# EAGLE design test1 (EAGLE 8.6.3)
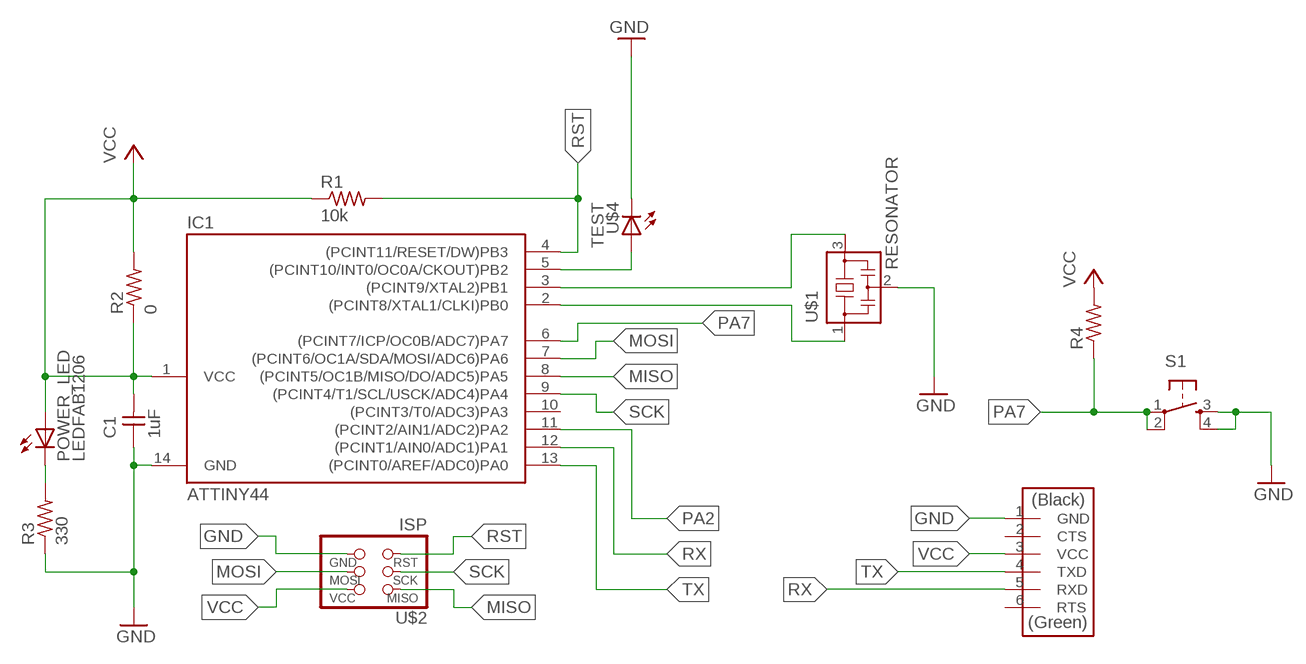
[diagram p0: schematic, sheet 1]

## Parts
C1  1uF  CAP-UNPOLARIZEDFAB  [C1206FAB]
FTDI  FTDI-SMD-HEADER  [1X06SMD]
IC1  ATTINY44  ATTINY44-SSU  [SOIC14]
POWER_LED  LEDFAB1206  [LED1206FAB]
R1  10k  RES-US1206FAB  [R1206FAB]
R2  0  RES-US1206FAB  [R1206FAB]
R3  330  RES-US1206FAB  [R1206FAB]
R4  RES-US1206FAB  [R1206FAB]
S1  6MM_SWITCH6MM_SWITCH  [6MM_SWITCH]
U$1  RESONATOR  [EFOBM]
U$2  ISP  AVRISPSMD  [2X03SMD]
U$4  TEST  LEDFAB1206  [LED1206FAB]

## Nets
GND: C1.1 FTDI.1(GND) IC1.14(GND) R3.1 S1.3(S) S1.4(S1) U$1.2 U$2.6(GND) U$4.2(C)
MISO: IC1.8((PCINT5/OC1B/MISO/DO/ADC5)PA5) U$2.1(MISO)
MOSI: IC1.7((PCINT6/OC1A/SDA/MOSI/ADC6)PA6) U$2.4(MOSI)
N$1: IC1.3((PCINT9/XTAL2)PB1) U$1.3
N$2: IC1.2((PCINT8/XTAL1/CLKI)PB0) U$1.1
N$4: POWER_LED.2(C) R3.2
N$6: IC1.5((PCINT10/INT0/OC0A/CKOUT)PB2) U$4.1(A)
PA2: IC1.11((PCINT2/AIN1/ADC2)PA2)
PA7: IC1.6((PCINT7/ICP/OC0B/ADC7)PA7) R4.1 S1.1(P) S1.2(P1)
RST: IC1.4((PCINT11/RESET/DW)PB3) R1.2 U$2.5(RST)
RX: FTDI.5(RXD) IC1.12((PCINT1/AIN0/ADC1)PA1)
SCK: IC1.9((PCINT4/T1/SCL/USCK/ADC4)PA4) U$2.3(SCK)
TX: FTDI.4(TXD) IC1.13((PCINT0/AREF/ADC0)PA0)
VCC: C1.2 FTDI.3(VCC) IC1.1(VCC) POWER_LED.1(A) R1.1 R2.1 R2.2 R4.2 U$2.2(VCC)
Unconnected: FTDI.2(CTS) FTDI.6(RTS) IC1.10((PCINT3/T0/ADC3)PA3)

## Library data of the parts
C1 = fab:CAP-UNPOLARIZED
FTDI = fab:FTDI-SMD-HEADER
IC1 = fab:ATTINY44
POWER_LED U$4 = fab:LED: LED
R1-R4 = fab:RES-US: Resistor (US Symbol)
S1 = fab:6MM_SWITCH: OMRON SWITCH
U$1 = fab:RESONATOR
U$2 = fab:AVRISP

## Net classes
0 default: width 0.508 mm, clearance 0.152 mm

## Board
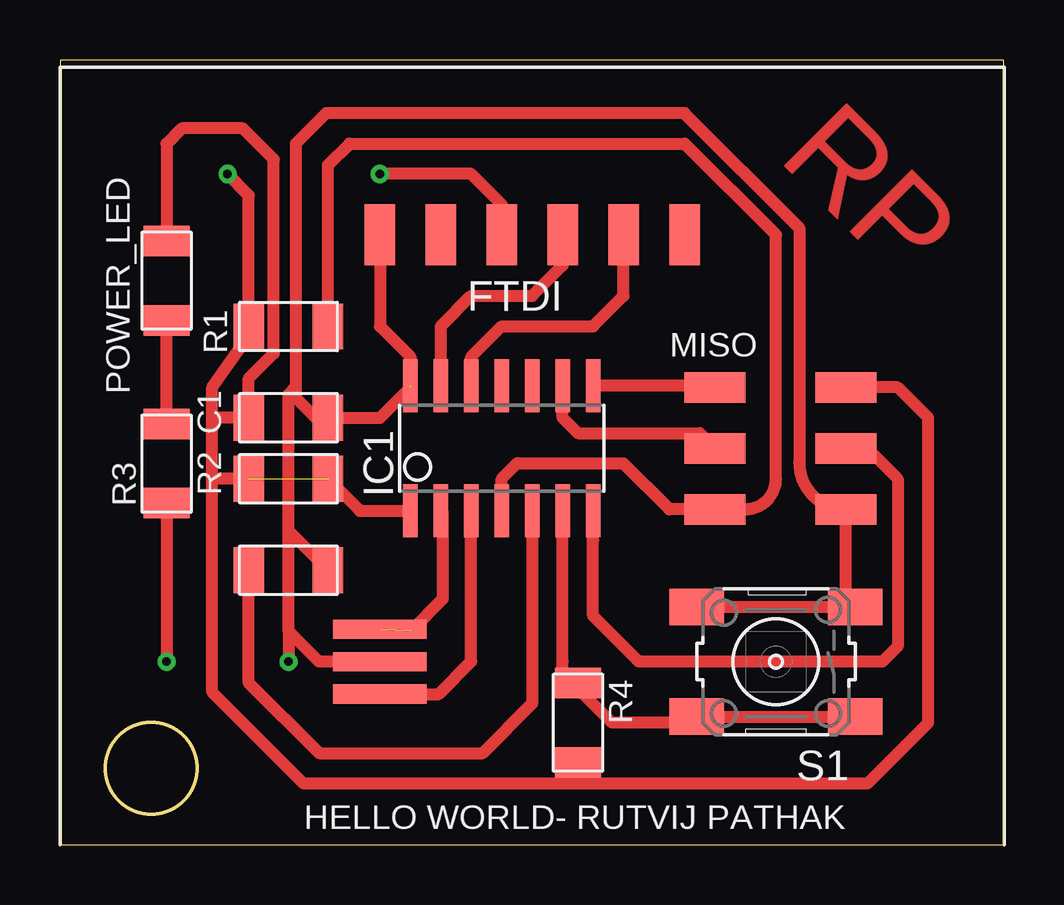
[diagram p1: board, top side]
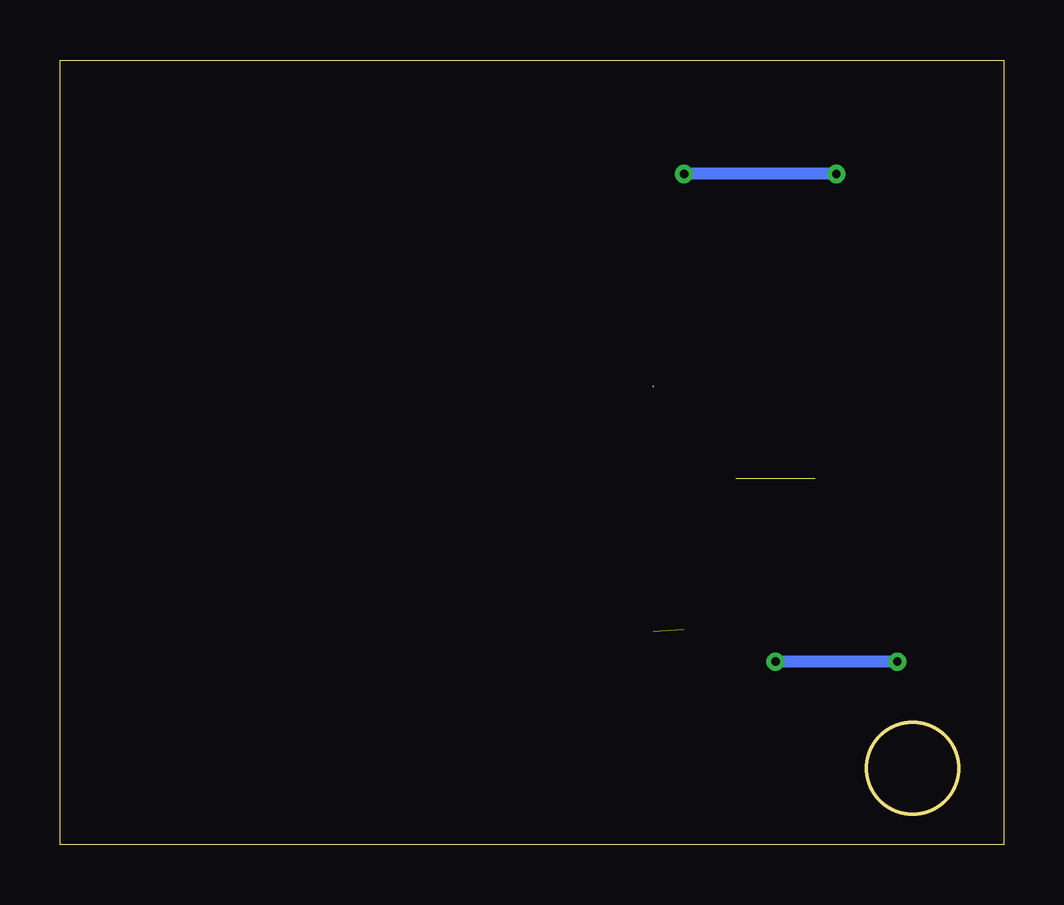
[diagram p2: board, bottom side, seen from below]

Size 39.35 x 32.69 mm. Coordinates in mm from the lower left corner, seen from the top.
Outline: 0,0 39.35,0 39.35,32.69 0,32.69 0,0
Outline: circle at 3.81,3.17 radius 1.91
Copper layers (1*16): Top 0.035mm / dielectric 1.5mm / Bottom 0.035mm
Design rules "default": minimum track width 6mil, minimum drill 0.35mm, track to track 6mil, track to pad 6mil, pad to pad 6mil, via to via 6mil, smd to smd 6mil, copper to edge 40mil, drill to drill 6mil, minimum pad ring 10mil, minimum via ring 8mil, stop-mask expansion 4mil, vias tented up to drill 0mil, thermal gap 10mil

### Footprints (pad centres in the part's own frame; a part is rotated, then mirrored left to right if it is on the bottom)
C1206FAB = smd 1.27 x 1.905: 1 -1.651,0; 2 1.651,0
1X06SMD = smd 2.54 x 1.27: 1 0,6.35; 2 0,3.81; 3 0,1.27; 4 0,-1.27; 5 0,-3.81; 6 0,-6.35
SOIC14 = smd 0.61 x 2.21: 1 -3.81,-2.603; 2 -2.54,-2.603; 3 -1.27,-2.603; 4 0,-2.603; 5 1.27,-2.603; 6 2.54,-2.603; 7 3.81,-2.603; 8 3.81,2.603; 9 2.54,2.603; 10 1.27,2.603; 11 0,2.603; 12 -1.27,2.603; 13 -2.54,2.603; 14 -3.81,2.603
LED1206FAB = smd 1.27 x 1.905: 1 -1.651,0; 2 1.651,0
R1206FAB = smd 1.27 x 1.905: 1 -1.651,0; 2 1.651,0
6MM_SWITCH = smd 2.286 x 1.524: 1 -3.302,2.286; 2 3.302,2.286; 3 -3.302,-2.286; 4 3.302,-2.286
EFOBM = smd 0.8 x 3.9: 1 -1.35,0; 2 0,0; 3 1.35,0
2X03SMD = smd 2.54 x 1.27: 1 -2.54,2.54; 2 2.92,2.54; 3 -2.54,0; 4 2.92,0; 5 -2.54,-2.54; 6 2.92,-2.54

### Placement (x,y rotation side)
C1  9.53,17.78 180 top
FTDI  19.68,25.4 90 top
IC1  18.41,16.51 0 top
POWER_LED  4.45,23.5 270 top
R1  9.53,21.59 0 top
R2  9.53,15.24 180 top
R3  4.45,15.88 90 top
R4  21.59,5.08 270 top
S1  29.84,7.62 180 top
U$1  13.34,7.62 270 top
U$2  29.84,16.51 0 top
U$4  9.53,11.43 0 top

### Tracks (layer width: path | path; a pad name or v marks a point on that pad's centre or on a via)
GND  (via drill 0.35)  (1 unrouted)
  Top 0.508: 9.82,19.05 9.82,29.21 11.1,30.48 26.04,30.48 30.82,25.7 30.82,15.92 arc90 U$2.6 | 9.82,19.05 9.82,18.62 11.18,17.27 C1.1 13.34,17.78 14.61,19.05 14.61,20.32 13.34,21.59 FTDI.1 | U$2.6 33.66,13.97 | U$1.2 10.79,7.62 9.53,8.89 | U$4.2 9.53,13.08 | 9.82,19.05 9.53,18.75 9.53,13.08 | 9.53,8.89 9.53,13.08 | R3.1 v4.45,7.62 | 9.53,8.89 v9.53,7.62 | S1.4 S1.3 32.77,10.29 U$2.6
  Bottom 0.508: v4.45,7.62 v9.53,7.62
MISO
  Top 0.508: U$2.1 27.24,19.11 IC1.8
MOSI
  Top 0.508: U$2.4 33.66,16.51 34.92,15.24 34.92,8.26 34.29,7.62 24.13,7.62 22.23,9.53 IC1.7 22.23,12.7
N$1
  Top 0.508: U$1.3 15.79,6.27 17.14,7.62 IC1.3
N$2  (1 unrouted)
  Top 0.508: IC1.2 15.96,13.83 15.96,10.24 14.61,8.89
N$4
  Top 0.508: R3.2 POWER_LED.2
N$6
  Top 0.508: U$4.1 7.87,6.73 10.79,3.81 17.63,3.81 19.68,5.87 IC1.5
PA7
  Top 0.152: R4.1 20.95,7.37 20.95,7.62
  Top 0.508: S1.1 S1.2 26.29,5.08 23.01,5.08 20.95,7.14 20.95,7.62 IC1.6
RST
  Top 0.508: R1.2 11.18,28.32 12.06,29.21 26.04,29.21 29.84,25.4 29.84,15.24 arc-90 28.57,13.97 U$2.5 25.4,13.97 23.5,15.88 19.1,15.88 19.07,15.9 18.41,15.24 IC1.4
RX
  Top 0.508: IC1.12 17.14,20.32 18.41,21.59 22.23,21.59 23.5,22.86 FTDI.5
SCK
  Top 0.508: IC1.9 20.95,17.78 21.59,17.14 26.67,17.14 U$2.3
TX
  Top 0.508: IC1.13 15.88,21.59 17.14,22.86 19.68,22.86 20.95,24.13 FTDI.4
VCC  (via drill 0.35)  (1 unrouted)
  Top 0.152: R4.2 21.59,2.54
  Top 0.508: U$2.2 33.66,19.05 | U$2.2 34.92,19.05 36.2,17.78 36.2,5.08 33.66,2.54 21.59,2.54 10.16,2.54 6.35,6.35 6.35,15.24 | 32.38,19.05 U$2.2 | R2.2 6.35,15.24 | FTDI.3 18.41,26.67 17.14,27.94 v13.34,27.94 | v6.99,27.94 7.87,27.05 R1.1 7.87,21.21 6.35,19.05 6.35,17.78 | 6.35,15.24 6.35,17.78 | R2.1 12.51,13.91 IC1.1 | 6.35,17.78 C1.2 7.87,19.43 8.91,20.47 8.91,28.55 7.62,29.84 5.08,29.84 4.45,29.21 POWER_LED.1
  Bottom 0.508: v6.99,27.94 v13.34,27.94

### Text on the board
Top: RP
tNames: MISO | HELLO WORLD- RUTVIJ PATHAK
